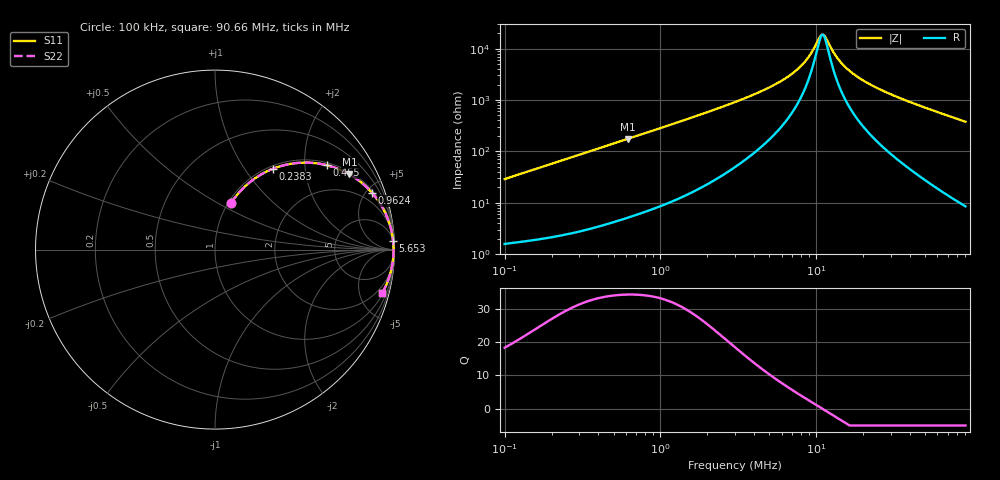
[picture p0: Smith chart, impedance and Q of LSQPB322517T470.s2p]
! LSQPB322517T470  S-PARAMETER MODEL  ( General Type )
! Model Generated by TAIYO YUDEN Corporation (http://www.ty-top.com)
! Version 2.0
! TAIYO YUDEN Control No. 100810NC14SB-FKC
! Copyright(c) 2008 TAIYO YUDEN CO.,LTD. All Rights Reserved.
! Product Description (link to TY-COMPAS)
! https://ds.yuden.co.jp/TYCOMPAS/or/detail?pn=LSQPB322517T470K&u=M
! Products Name : Inductors
! Characteristics :
!  Inductance : 47 uH , SRF(min) : 7.0 MHz , DC Resistance(max) : 1.2 Ohm
!  Rated Current : Saturation :420 mA , Temp Rise : 390 mA (40 degC)
!  Case Size : 3.2 x 2.5 / 0.126 x 0.098 [mm/inch] , Thickness : 1.7 / 0.068 [mm/inch]
!  (Conditions: Temperature = 25 degC , DC Bias Current/Voltage = 0A / 0V)
! External Node Assignments :
!  1  o---GGG---o  2
! GND o---------o GND
! Frequency Range : 0.1MHz  -  90.659724MHz  [ 402 STEP ]
# MHz S RI R 50
! Freq[MHz].  S11 Real  S11 Imag  S21 Real  S21 Imag  S12 Real  S12 Imag  S22 Real  S22 Imag
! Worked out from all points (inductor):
!   401 points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, 100 kHz to 90.66 MHz, reference 50 ohm
!   read as one part in series: L = 45.8 uH near 103.5 kHz
!   highest Q = 34.2 at 618.2 kHz (marker M1), where L = 45.2 uH
!   self-resonance near 10.98 MHz
!   S11 on the Smith chart (normalised r, x): 100 kHz: 1.03, +0.58; 238.3 kHz: 1.05, +1.36; 455 kHz: 1.08, +2.59; 962.4 kHz: 1.16, +5.46; 5.653 MHz: 6, +42; 90.66 MHz: 1.17, -7.56
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0.1  0.0893 0.259  0.9107 -0.259  0.9107 -0.259  0.0893 0.259
0.15568  0.177 0.3611  0.823 -0.3611  0.823 -0.3611  0.177 0.3611
0.238271  0.323 0.4506  0.677 -0.4506  0.677 -0.4506  0.323 0.4506
0.312872  0.4453 0.4814  0.5547 -0.4814  0.5547 -0.4814  0.4453 0.4814
0.455014  0.6227 0.4701  0.3773 -0.4701  0.3773 -0.4701  0.6227 0.4701
0.618171  0.7486 0.4194  0.2514 -0.4194  0.2514 -0.4194  0.7486 0.4194
0.962366  0.8745 0.3166  0.1255 -0.3166  0.1255 -0.3166  0.8745 0.3166
0.97889  0.8781 0.3125  0.1219 -0.3125  0.1219 -0.3125  0.8781 0.3125
1.603786  0.9483 0.2046  0.0517 -0.2046  0.0517 -0.2046  0.9483 0.2046
3.062674  0.9829 0.105  0.0171 -0.105  0.0171 -0.105  0.9829 0.105
5.652857  0.9925 0.0458  0.00754 -0.0458  0.00754 -0.0458  0.9925 0.0458
7.679831  0.9941 0.0235  0.00589 -0.0235  0.00589 -0.0235  0.9941 0.0235
8.651799  0.9944 0.0155  0.00555 -0.0155  0.00555 -0.0155  0.9944 0.0155
9.420503  0.9946 0.00993  0.0054 -0.00993  0.0054 -0.00993  0.9946 0.00993
10.61277  0.9947 0.00223  0.00529 -0.00223  0.00529 -0.00223  0.9947 0.00223
11.16888  0.9947 -0.00106  0.00528 0.00106  0.00528 0.00106  0.9947 -0.00106
11.55571  0.9947 -0.00325  0.00529 0.00325  0.00529 0.00325  0.9947 -0.00325
13.46909  0.9946 -0.0132  0.00544 0.0132  0.00544 0.0132  0.9946 -0.0132
15.96885  0.9941 -0.0246  0.00587 0.0246  0.00587 0.0246  0.9941 -0.0246
20.61469  0.9929 -0.0431  0.00714 0.0431  0.00714 0.0431  0.9929 -0.0431
29.47413  0.9892 -0.0739  0.0108 0.0739  0.0108 0.0739  0.9892 -0.0739
90.65972  0.9299 -0.2443  0.0701 0.2443  0.0701 0.2443  0.9299 -0.2443
